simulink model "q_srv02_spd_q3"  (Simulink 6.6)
settings: Solver=ode1  StartTime=0.0  StopTime=inf  FixedStep=0.002  RelTol=1e-3  AbsTol=1e-6
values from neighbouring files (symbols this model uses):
  a = 10^(-21/20)    (= 0.0891250938134)    [d_lag_q3.m]    (also in d_lead.m = (1+sin(phi_m)) / (1-sin(phi_m)); setup_srv02_exp03_spd.m = 1)
  bsp = 0    [setup_srv02_exp03_spd.m]
  IMAX_AMP = 0    [config_srv02.m]
  K_ENC = 0    [config_srv02.m]
  K_POT = -(352 * pi / 180 / 10)    (= -0.614355896702)    [config_srv02.m]
  K_TACH = -(1000 * 2 * pi / 60 / 1.5 / Kg)    [config_srv02.m]
  Kc = 10^(e_ss_meas/e_ss_min/20)    (= 2.14783047413)    [d_lag_q3.m]    (also in d_lead.m = 53.0884444231; setup_srv02_exp03_spd.m = 0)
  ki = wn^2*tau/K    [d_pi_design.m]    (also in setup_srv02_exp03_spd.m = 0; d_i_design.m = -( -AmpMax + kp * e_ss ) / ti / e_ss; setup_srv02_exp02_pos.m = 0)
  kp = (-1+2*zeta*wn*tau)/K    [d_pi_design.m]    (also in setup_srv02_exp03_spd.m = 0; d_pv_design.m = wn^2/K*tau; setup_srv02_exp02_pos.m = 0)
  T = 10 / (wg_des * a)    [d_lag_q3.m]    (also in d_lead.m = 1 / (w_m * sqrt(a)); setup_srv02_exp03_spd.m = 1)
  VMAX_DAC = 10    [setup_srv02_exp03_spd.m]    (also in setup_srv02_exp01_mdl.m; setup_srv02_exp02_pos.m)
  wcf_e = 2 * pi * 63.0    (= 395.840674352)    [setup_srv02_exp03_spd.m]    (also in setup_srv02_exp01_mdl.m = 157.079632679; setup_srv02_exp02_pos.m = 314.159265359)
  zetaf_e = 0.9    [setup_srv02_exp03_spd.m]    (also in setup_srv02_exp01_mdl.m; setup_srv02_exp02_pos.m)
undefined symbols (not defined in the file or in its folder): HIL, qc_get_step_size, square
libraries: quarc_library x5, simulink x3

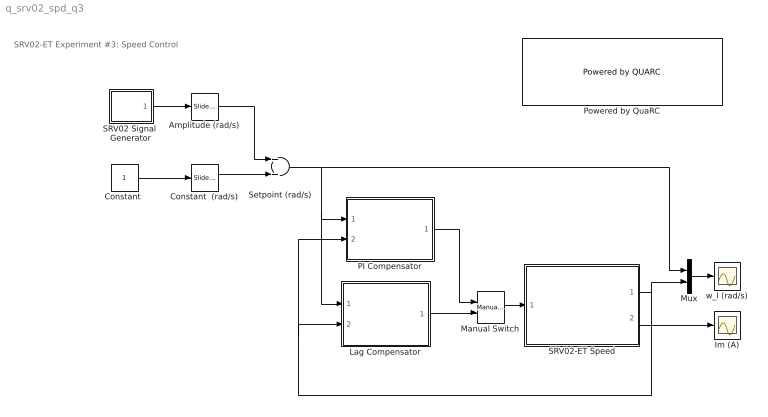
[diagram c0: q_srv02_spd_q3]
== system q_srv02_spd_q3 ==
  note: SRV02-ET Experiment #3: Speed Control
  Amplitude (rad/s) : simulink/Math Operations/Slider Gain  SystemSampleTime=-1  low=0  gain=2.5  high=10
  "Constant " : Constant
  Constant  (rad/s) : simulink/Math Operations/Slider Gain  SystemSampleTime=-1  low=0  gain=5  high=10
  Im (A) : Scope
  Lag Compensator : Subsystem
  Manual Switch : simulink/Signal Routing/Manual Switch  SystemSampleTime=-1  sw=1  action=0  varsize=off
  Mux : Mux  Inputs=2
  PI Compensator : Subsystem
  Powered by QuaRC : quarc_library/Logos/Powered by QUARC  SystemSampleTime=-1
  SRV02 Signal  Generator : Subsystem  mask(QET Signal Generator){sig_type=square, a=1, f=0.4}
      mask prompts: sig_type "Signal Type"; a "Amplitude"; f "Frequency (Hz)"
      mask help: Generates a square, triangular, or sinusoidal waveform of a specified amplitude and frequency.
  SRV02-ET Speed : Subsystem
  Setpoint (rad/s) : Sum  OutScaling=2^-10
  w_l (rad/s) : Scope
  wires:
  Setpoint (rad/s)/1 -> Mux/1, PI Compensator/1(wd (rad/s)), Lag Compensator/1(wd (rad/s))
  SRV02-ET Speed/2(Im (A)) -> Im (A)/1
  Mux/1 -> w_l (rad/s)/1
  SRV02 Signal  Generator/1(out) -> Amplitude (rad/s)/1
  Amplitude (rad/s)/1 -> Setpoint (rad/s)/1
  "Constant "/1 -> Constant  (rad/s)/1
  SRV02-ET Speed/1(omega_l (rad/s)) -> PI Compensator/2(wl (rad)), Lag Compensator/2(wl (rad/s)), Mux/2
  PI Compensator/1(I_ref (A)) -> Manual Switch/1
  Lag Compensator/1(I_ref (A)) -> Manual Switch/2
  Manual Switch/1 -> SRV02-ET Speed/1(I_ref (A))
  Constant  (rad/s)/1 -> Setpoint (rad/s)/2

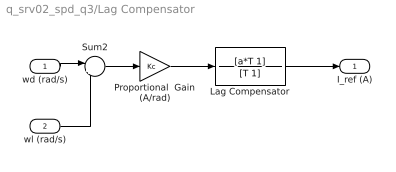
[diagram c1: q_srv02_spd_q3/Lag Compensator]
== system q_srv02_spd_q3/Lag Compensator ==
  wd (rad/s) : Inport
  wl (rad/s) : Inport  Port=2
  Lag Compensator : TransferFcn  Numerator=[a*T 1]  Denominator=[T 1]
  Proportional  Gain (A/rad) : Gain  Gain=Kc
  Sum2 : Sum  Inputs=|+-
  I_ref (A) : Outport
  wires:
  wl (rad/s)/1 -> Sum2/2
  wd (rad/s)/1 -> Sum2/1
  Sum2/1 -> Proportional  Gain (A/rad)/1
  Proportional  Gain (A/rad)/1 -> Lag Compensator/1
  Lag Compensator/1 -> I_ref (A)/1

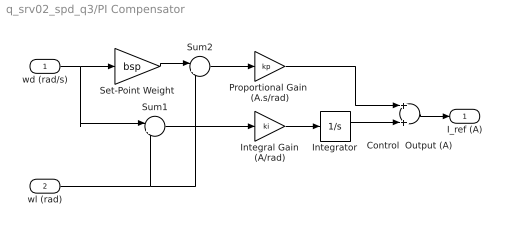
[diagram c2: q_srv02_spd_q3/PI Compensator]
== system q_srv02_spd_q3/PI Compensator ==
  wd (rad/s) : Inport
  wl (rad) : Inport  Port=2
  Control  Output (A) : Sum  OutScaling=2^-10
  Integral Gain (A/rad) : Gain  Gain=ki
  Integrator : Integrator  UpperSaturationLimit=10  LowerSaturationLimit=-10
  Proportional Gain  (A.s/rad) : Gain  Gain=kp
  Set-Point Weight : Gain  Gain=bsp
  Sum1 : Sum  Inputs=|+-
  Sum2 : Sum  Inputs=|+-
  I_ref (A) : Outport
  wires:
  wl (rad)/1 -> Sum2/2, Sum1/2
  Control  Output (A)/1 -> I_ref (A)/1
  wd (rad/s)/1 -> Sum1/1, Set-Point Weight/1
  Sum2/1 -> Proportional Gain  (A.s/rad)/1
  Set-Point Weight/1 -> Sum2/1
  Proportional Gain  (A.s/rad)/1 -> Control  Output (A)/1
  Integrator/1 -> Control  Output (A)/2
  Integral Gain (A/rad)/1 -> Integrator/1
  Sum1/1 -> Integral Gain (A/rad)/1

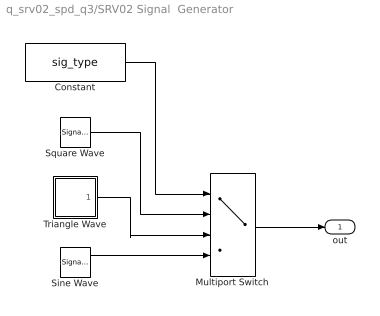
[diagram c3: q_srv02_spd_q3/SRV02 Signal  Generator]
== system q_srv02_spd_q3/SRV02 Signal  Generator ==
  Constant : Constant  Value=sig_type
  Multiport Switch : MultiPortSwitch  Inputs=3
  Sine Wave : SignalGenerator  Amplitude=a  Frequency=f
  Square Wave : SignalGenerator  WaveForm=square  Amplitude=a  Frequency=f
  Triangle Wave : Subsystem
  out : Outport
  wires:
  Constant/1 -> Multiport Switch/1
  Multiport Switch/1 -> out/1
  Sine Wave/1 -> Multiport Switch/4
  Triangle Wave/1(out) -> Multiport Switch/3
  Square Wave/1 -> Multiport Switch/2

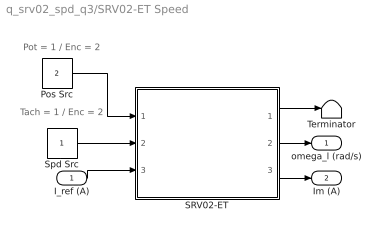
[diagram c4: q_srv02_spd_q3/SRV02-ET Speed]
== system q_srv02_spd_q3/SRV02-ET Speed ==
  note: Pot = 1 / Enc = 2
  note: Tach = 1 / Enc = 2
  I_ref (A) : Inport
  Pos Src : Constant  Value=2
  SRV02-ET : Subsystem
  Spd Src : Constant
  Terminator : Terminator
  omega_l (rad/s) : Outport
  Im (A) : Outport  Port=2
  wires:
  Pos Src/1 -> SRV02-ET/1(pos src)
  SRV02-ET/1(theta_l (rad)) -> Terminator/1
  SRV02-ET/2(omega_l (rad/s)) -> omega_l (rad/s)/1
  I_ref (A)/1 -> SRV02-ET/3(I_ref (A))
  SRV02-ET/3(Im (A)) -> Im (A)/1
  Spd Src/1 -> SRV02-ET/2(spd src)

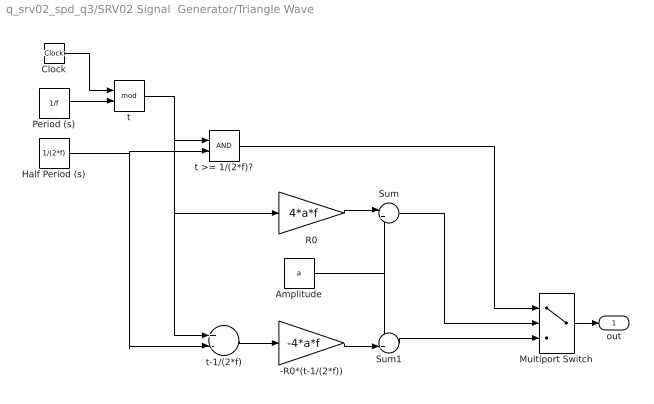
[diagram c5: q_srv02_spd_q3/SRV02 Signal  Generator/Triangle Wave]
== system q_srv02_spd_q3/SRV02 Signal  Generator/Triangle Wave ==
  -R0*(t-1/(2*f)) : Gain  Gain=-4*a*f
  Amplitude : Constant  Value=a
  Clock : Clock
  Half Period (s) : Constant  Value=1/(2*f)
  Multiport Switch : MultiPortSwitch  Inputs=2  zeroidx=on
  Period (s) : Constant  Value=1/f
  R0 : Gain  Gain=4*a*f
  Sum : Sum  Inputs=|+-
  Sum1 : Sum  Inputs=++|
  t : Math  Operator=mod
  t >= 1/(2*f)? : RelationalOperator  LogicOutDataTypeMode=Boolean
  t-1/(2*f) : Sum  Inputs=+-  OutScaling=2^-10
  out : Outport
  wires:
  Multiport Switch/1 -> out/1
  Clock/1 -> t/1
  Period (s)/1 -> t/2
  t/1 -> t >= 1/(2*f)?/1, R0/1, t-1/(2*f)/1
  Half Period (s)/1 -> t >= 1/(2*f)?/2, t-1/(2*f)/2
  t-1/(2*f)/1 -> -R0*(t-1/(2*f))/1
  R0/1 -> Sum/1
  Amplitude/1 -> Sum/2, Sum1/1
  -R0*(t-1/(2*f))/1 -> Sum1/2
  t >= 1/(2*f)?/1 -> Multiport Switch/1
  Sum/1 -> Multiport Switch/2
  Sum1/1 -> Multiport Switch/3

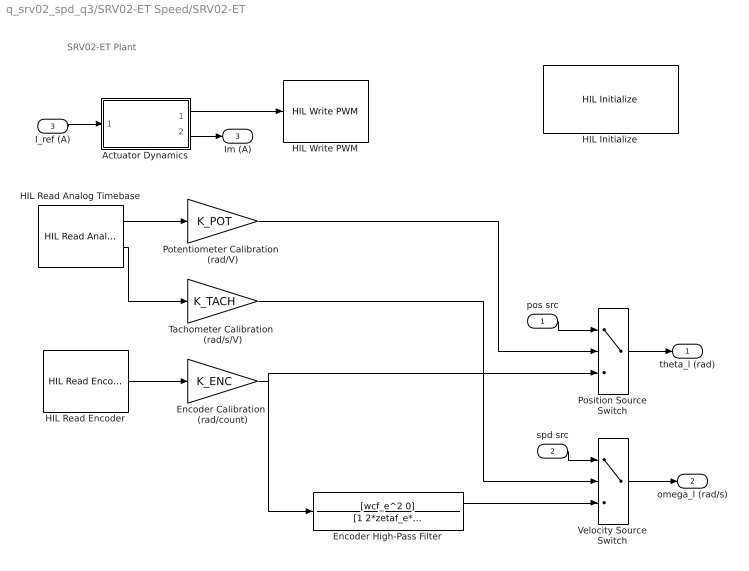
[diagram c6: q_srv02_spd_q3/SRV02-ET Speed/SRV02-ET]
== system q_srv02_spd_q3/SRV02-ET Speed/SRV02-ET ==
  note: SRV02-ET Plant
  pos src : Inport
  spd src : Inport  Port=2
  I_ref (A) : Inport  Port=3
  Actuator Dynamics : Subsystem
  Encoder Calibration  (rad/count) : Gain  Gain=K_ENC
  Encoder High-Pass Filter : TransferFcn  Numerator=[wcf_e^2 0]  Denominator=[1 2*zetaf_e*wcf_e wcf_e^2]
  HIL Initialize : quarc_library/Data Acquisition/Generic/Configuration/HIL Initialize  object_name=HIL-1  board_type=q3_controlpaq_fw  board_number=0  exclusive=off  active=on  hardware_clocks=[]  clock_modes=[]  set_clock_params_at_start=off  set_clock_params_at_switch_in=off  analog_input_channels=0:1  analog_input_maximums=10  analog_input_minimums=-10  set_analog_input_params_at_start=off  set_analog_input_params_at_switch_in=off  analog_output_channels=[]  analog_output_maximums=[]  analog_output_minimums=[]  initial_analog_outputs=[]  final_analog_outputs=[]  watchdog_analog_outputs=0  set_analog_output_params_at_start=off  set_analog_output_params_at_switch_in=off  set_analog_outputs_at_start=off  set_analog_outputs_at_switch_in=off  set_analog_outputs_at_terminate=off  set_analog_outputs_at_switch_out=off  set_analog_outputs_on_watchdog=off  digital_input_channels=[]  digital_output_channels=[]  digital_output_configuration=[]  initial_digital_outputs=[]  final_digital_outputs=[]  watchdog_digital_outputs=0  set_digital_output_params_at_start=off  set_digital_output_params_at_switch_in=off  set_digital_outputs_at_start=off  set_digital_outputs_at_switch_in=off  set_digital_outputs_at_terminate=off  set_digital_outputs_at_switch_out=off  set_digital_outputs_on_watchdog=off  encoder_channels=0:2  quadrature=[]  encoder_filter_frequency=[]  initial_encoder_counts=0  set_encoder_params_at_start=off  set_encoder_params_at_switch_in=off  set_encoder_counts_at_start=on  set_encoder_counts_at_switch_in=off  pwm_channels=0:2  pwm_modes=[]  pwm_frequency=[]  pwm_configuration=[]  pwm_alignment=[]  pwm_polarity=[]  pwm_leading_deadband=[]  pwm_trailing_deadband=[]  initial_pwm_outputs=0  final_pwm_outputs=0  watchdog_pwm_outputs=0  set_pwm_params_at_start=off  set_pwm_params_at_switch_in=off  set_pwm_outputs_at_start=on  set_pwm_outputs_at_switch_in=off  set_pwm_outputs_at_terminate=on  set_pwm_outputs_at_switch_out=off  set_pwm_outputs_on_watchdog=off  other_output_channels=[]  initial_other_outputs=[]  final_other_outputs=[]  watchdog_other_outputs=0  set_other_outputs_at_start=off  set_other_outputs_at_switch_in=off  set_other_outputs_at_terminate=off  set_other_outputs_at_switch_out=off  set_other_outputs_on_watchdog=off
  HIL Read Analog Timebase : quarc_library/Data Acquisition/Generic/Timebases/HIL Read Analog Timebase  Tag=unassigned  object_name=HIL-1  clock=0  channels=[0:1]  samples_in_buffer=max(ceil(1/qc_get_step_size), 1)  active=on  vector_output=off
  HIL Read Encoder : quarc_library/Data Acquisition/Generic/Immediate I//O/HIL Read Encoder  Tag=unassigned  object_name=HIL-1  channels=0  sample_time=qc_get_step_size  active=on  vector_output=off  data_type_mode=Inherit via back propagation  data_type=double
  HIL Write PWM : quarc_library/Data Acquisition/Generic/Immediate I//O/HIL Write PWM  object_name=HIL-1  channels=0  sample_time=-1  active=off  vector_input=off
  Position Source Switch : MultiPortSwitch  Inputs=2
  Potentiometer Calibration  (rad/V) : Gain  Gain=K_POT
  Tachometer Calibration  (rad/s/V) : Gain  Gain=K_TACH
  Velocity Source Switch : MultiPortSwitch  Inputs=2
  theta_l (rad) : Outport  InitialOutput=0
  omega_l (rad/s) : Outport  Port=2  InitialOutput=0
  Im (A) : Outport  Port=3  InitialOutput=0
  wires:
  Position Source Switch/1 -> theta_l (rad)/1
  Potentiometer Calibration  (rad/V)/1 -> Position Source Switch/2
  pos src/1 -> Position Source Switch/1
  HIL Read Analog Timebase/1 -> Potentiometer Calibration  (rad/V)/1
  HIL Read Analog Timebase/2 -> Tachometer Calibration  (rad/s/V)/1
  Actuator Dynamics/1(Vdaq (V)) -> HIL Write PWM/1
  Tachometer Calibration  (rad/s/V)/1 -> Velocity Source Switch/2
  Encoder Calibration  (rad/count)/1 -> Position Source Switch/3, Encoder High-Pass Filter/1
  I_ref (A)/1 -> Actuator Dynamics/1(I_ref (A))
  Actuator Dynamics/2(Im (A)) -> Im (A)/1
  Velocity Source Switch/1 -> omega_l (rad/s)/1
  spd src/1 -> Velocity Source Switch/1
  Encoder High-Pass Filter/1 -> Velocity Source Switch/3
  HIL Read Encoder/1 -> Encoder Calibration  (rad/count)/1

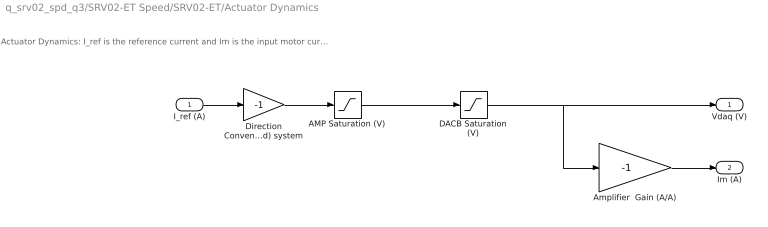
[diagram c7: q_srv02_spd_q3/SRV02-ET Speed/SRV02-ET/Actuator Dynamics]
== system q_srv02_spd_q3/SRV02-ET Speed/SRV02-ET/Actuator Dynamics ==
  note: Actuator Dynamics: I_ref is the reference current and Im is the input motor current after going through the DACB and amplifier limitiations.
  I_ref (A) : Inport
  AMP Saturation (V) : Saturate  UpperLimit=IMAX_AMP  LowerLimit=-IMAX_AMP
  Amplifier  Gain (A/A) : Gain  Gain=-1
  DACB Saturation (V) : Saturate  UpperLimit=VMAX_DAC  LowerLimit=-VMAX_DAC
  Direction Convention: (Right-Hand) system : Gain  Gain=-1
  Vdaq (V) : Outport
  Im (A) : Outport  Port=2
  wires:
  I_ref (A)/1 -> Direction Convention: (Right-Hand) system/1
  AMP Saturation (V)/1 -> DACB Saturation (V)/1
  DACB Saturation (V)/1 -> Amplifier  Gain (A/A)/1, Vdaq (V)/1
  Amplifier  Gain (A/A)/1 -> Im (A)/1
  Direction Convention: (Right-Hand) system/1 -> AMP Saturation (V)/1
